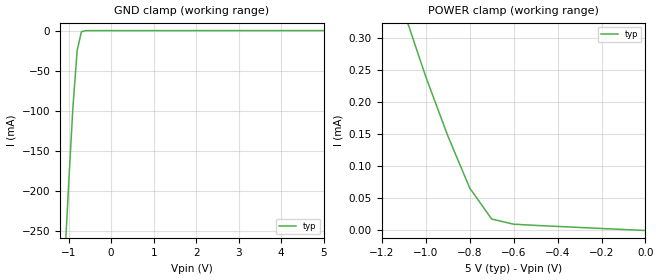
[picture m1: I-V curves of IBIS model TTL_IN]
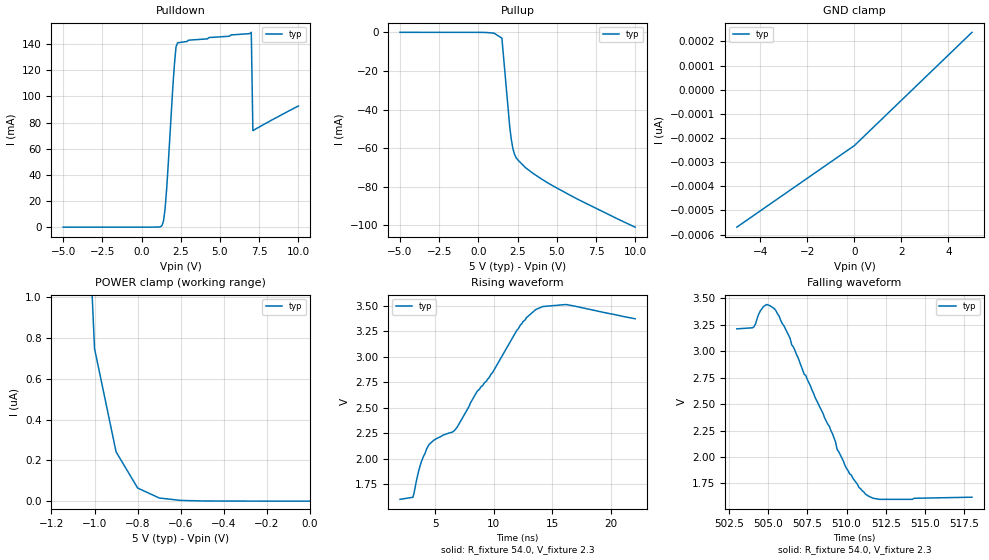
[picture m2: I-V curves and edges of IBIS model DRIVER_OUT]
|   Texas Instruments Incorporated
|   Data Transmissions Products
|   IBIS Model for SN75LBC174A
|   20P SOIC Package
[IBIS Ver]   3.2
[Comment char]   |_char
[File name]   lbc174adw.ibs
[File Rev]   2.0
[Date]   16Jan01
[Source]   File originated at Texas Instruments Incorporated.
   Data Transmission Products Group. All data based on
   Bench Measurements.
[Notes]
[Disclaimer]
(C) Copyright Texas Instruments Incorporated 2001
   All rights reserved
  Texas Instruments Incorporated hereby grants the user of this IBIS
model a non-exclusive, nontransferable license to use this IBIS model
under the following terms.  Before using this IBIS model, the user
should read this license.  If the user does not accept these terms,
the IBIS model should be returned to Texas Instruments within 30 days.
  The user is granted this license only to use the IBIS model and
is not granted rights to sell, load, rent, lease or license the IBIS
model in whole or in part, or in modified form to anyone other than
user.  User may modify the IBIS model to suit its specific applications
but rights to derivative works and such modifications shall belong to
Texas Instruments.
  This IBIS model is provided on an "AS IS" basis and Texas Instruments
makes absolutely no warranty with respect to the information contained
herein.  TEXAS INSTRUMENTS DISCLAIMS AND CUSTOMER WAIVES ALL WARRANTIES,
EXPRESS OR IMPLIED, INCLUDING WARRANTIES OF MERCHANTABILITY OR FITNESS
FOR A PARTICULAR PURPOSE. The entire risk as to quality and performance
is with the Customer. ACCORDINGLY, IN NO EVENT SHALL THE COMPANY BE LIABLE
FOR ANY DAMAGES, WHETHER IN CONTRACT OR TORT,INCLUDING ANY LOST PROFITS
OR OTHER INCIDENTAL, CONSEQUENTIAL, EXEMPLARY, OR PUNITIVE DAMAGES ARISING
OUT OF THE USE OR APPLICATION OF THE IBIS model provided in this package.
Further, Texas Instruments reserves the right to discontinue or make changes
without notice to any product herein to improve reliability, function, or
design. Texas Instruments does not convey any license under patent rights
or any other intellectual property rights, including those of third parties.
Contact Texas Instruments at ATTN:DATA TRANSMISSIONS
[Copyright]   Copyright 2001, Texas Instruments, All Rights Reserved
[Component]   SN75LBC174ADW
[Manufacturer]  Texas Instruments Incorporated
[Package]
|   typ   min   max
R_pkg   0.038   0.034   0.045
L_pkg   5.130nH   4.110nH   6.349nH
C_pkg   0.731pF   0.530pF   0.868pF
[Pin]   signal_name   model_name   R_pin   L_pin   C_pin
1   1A   TTL_IN   0.042   6.336n   0.865p
2   1Y   DRIVER_OUT   0.043   5.542n   0.867p
3   NC   NC
4   1Z   DRIVER_OUT   0.034   4.377n   0.591p
5   1,2EN   TTL_IN   0.036   4.130n   0.533p
6   2Z   DRIVER_OUT   0.035   4.111n   0.530p
7   NC   NC
8   2Y   DRIVER_OUT   0.034   4.634n   0.726p
9   2A   TTL_IN   0.040   5.518n   0.865p
10   GND   GND   0.043   6.349n   0.866p
11   3A   TTL_IN   0.041   6.281n   0.861p
12   3Y   DRIVER_OUT   0.045   5.561n   0.868p
13   NC   NC
14   3Z   DRIVER_OUT   0.035   4.414n   0.596p
15   3,4EN   TTL_IN   0.035   4.110n   0.533p
16   4Z   DRIVER_OUT   0.036   4.130n   0.533p
17   NC   NC
18   4Y   DRIVER_OUT   0.034   4.714n   0.731p
19   4A   TTL_IN   0.043   5.569n   0.868p
20   VCC   POWER   0.042   6.308n   0.864p
[Diff_pin]   inv_pin   vdiff   tdelay_typ   tdelay_min   tdelay_max
| The 'xY' pin is Diff_pin and the 'xZ' pin is the inv_pin
2   4   NA   0 0 0
8   6   NA   0 0 0
12   14   NA   0 0 0
18   16   NA   0 0 0
| Models and submodels in the file (2): TTL_IN (Input), DRIVER_OUT (3-state)
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|   TTL Input Model
[Model]   TTL_IN
Model_type   Input
|Signals   1,2EN,3,4EN,1A,2A,3A,4A
Vinh = 2.0
Vinl = 0.8
|   typ   min   max
C_comp   1.0pF   NA   NA
|   typ   min   max
[Temperature Range]   25.0   NA   NA
[Voltage range]   5.0V   4.75V   5.25V
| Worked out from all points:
|   GND clamp passes 1 mA (typ) near -0.67 V on its own axis
[GND_clamp]
|   Voltage   I(typ)   I(min)   I(max)
-5V       -4.21A     NA         NA
-2V       -1.22A     NA         NA
-1V       -192mA     NA         NA
-900mV    -96.1mA    NA         NA
-800mV    -24.8mA    NA         NA
-700mV    -1.47mA    NA         NA
-500mV    -28.2uA    NA         NA
5V        11.6pA     NA         NA
[Power_clamp]
| Note that the[POWER_clamp]voltage table is referenced to Vcc
| and is calculated using Vtable=Vcc - Vmeasured.
|   Voltage   I(typ)   I(min)   I(max)
-5V       4.42mA     NA         NA
-2V       1.26mA     NA         NA
-1V       240uA      NA         NA
-900mV    148uA      NA         NA
-800mV    66.3uA     NA         NA
-700mV    17.8uA     NA         NA
-600mV    9.8uA      NA         NA
0V        11.6pA     NA         NA
|   Driver Output Model
[Model]   DRIVER_OUT
Model_type   3-state
| Signals   1Y,1Z,2Y,2Z,3Y,3Z,4Y,4Z
Vmeas = 2.3V   |Reference voltage for timing measurements
Cref = 50pF   |Timing specification test load capacitance value
Rref = 54   |Note: 54 Ohm load; single ended configuration
|   typ   min   max
C_comp   1.0pF   NA   NA
|   typ   min   max
[Temperature Range]   25.0   NA   NA
[Voltage range]   5.0V   4.75V   5.25V
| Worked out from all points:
|   slope of the pulldown table from 0 to 0.75 V, typ, clamps not added: 18.8 kohm
|   slope of the pullup table from 0 to 0.75 V, typ, clamps not added: 3.08 kohm
|   rising waveform, R_fixture 54.0, V_fixture 2.3: 20-80 % time 7ns typ, NA min, NA max; typ from 1.6 V to 3.37 V
|   falling waveform, R_fixture 54.0, V_fixture 2.3: 20-80 % time 2.84ns typ, NA min, NA max; typ from 3.21 V to 1.62 V
[Pulldown]
|   Voltage   I(typ)   I(min)   I(max)
-5V       -560pA     NA         NA
1.3V      1.13mA     NA         NA
1.4V      4.65mA     NA         NA
1.5V      13.9mA     NA         NA
1.6V      29mA       NA         NA
2V        108mA      NA         NA
2.1V      125mA      NA         NA
2.2V      138mA      NA         NA
2.3V      141mA      NA         NA
7V        149mA      NA         NA
7.1V      73.8mA     NA         NA
10V       92.6mA     NA         NA
[Pullup]
|   Voltage   I(typ)   I(min)   I(max)
| Note that the[Pullup]voltage table is referenced to Vcc
| and is calculated using Vtable=Vcc - Vmeasured.
-5V       16.6uA     NA         NA
500mV     -60.3uA    NA         NA
1V        -426uA     NA         NA
1.5V      -3.01mA    NA         NA
2V        -49mA      NA         NA
2.1V      -55.5mA    NA         NA
2.2V      -60.2mA    NA         NA
2.4V      -64.9mA    NA         NA
3V        -70.1mA    NA         NA
4.5V      -78.4mA    NA         NA
6.5V      -87.2mA    NA         NA
10V       -101mA     NA         NA
| Output in High Impedance (off)
[GND_clamp]
|   Voltage   I(typ)   I(min)   I(max)
-5V       -569pA     NA         NA
0V        -231pA     NA         NA
5V        238pA      NA         NA
[POWER_clamp]
|   Voltage   I(typ)   I(min)   I(max)
| Note that the [POWER_clamp] voltage table is referenced to Vcc
| and is calculated using Vtable = Vcc - Vmeasured.
| Outputs in Tri-state.
-5V       16.6uA     NA         NA
-1.5V     12.7uA     NA         NA
-1V       749nA      NA         NA
-900mV    242nA      NA         NA
-800mV    64.6nA     NA         NA
-700mV    15.6nA     NA         NA
-600mV    3.78nA     NA         NA
0V        238pA      NA         NA
[Ramp]
|   typ   min   max
dV/dt_r   1.77v/7ns   NA   NA
dV/dt_f   1.60v/3.2ns   NA   NA
R_load = 54ohm  | Note: The measurement is single-ended with respect
|   to ground.
[Rising Waveform]
R_fixture = 54.0
V_fixture = 2.3
C_fixture = 0p
L_fixture = 0n
|   V(typ)   V(min)   V(max)
2ns       1.6V       NA         NA
3.1ns     1.62V      NA         NA
3.8ns     1.96V      NA         NA
4.5ns     2.14V      NA         NA
6.7ns     2.28V      NA         NA
9.9ns     2.84V      NA         NA
12ns      3.26V      NA         NA
13.6ns    3.46V      NA         NA
16.2ns    3.51V      NA         NA
22.1ns    3.37V      NA         NA
[Falling Waveform]
R_fixture = 54.0
V_fixture = 2.3
C_fixture = 0p
L_fixture = 0n
|   V(typ)   V(min)   V(max)
503ns     3.21V      NA         NA
504.1ns   3.23V      NA         NA
504.5ns   3.38V      NA         NA
504.9ns   3.44V      NA         NA
505.4ns   3.4V       NA         NA
508.9ns   2.29V      NA         NA
509.4ns   2.07V      NA         NA
511.2ns   1.65V      NA         NA
512.1ns   1.6V       NA         NA
518ns     1.62V      NA         NA
